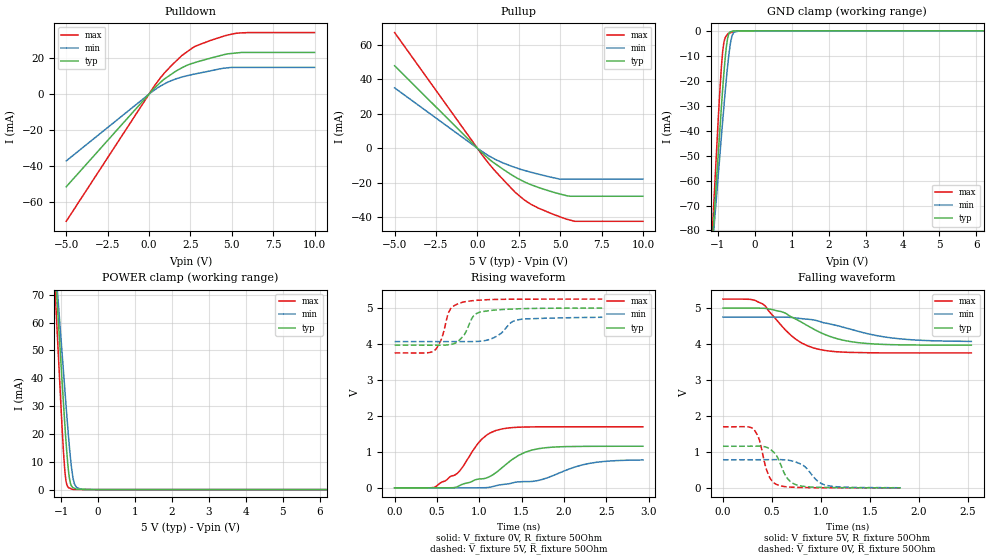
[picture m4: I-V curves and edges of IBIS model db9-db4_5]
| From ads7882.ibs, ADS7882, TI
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|   db9-db4_5 Model
[Model]   db9-db4_5
Model_type   3-state
Polarity   Non-Inverting
Enable   Active-Low
Vmeas = 2.5
Vref = 2.5
Cref = 20pF
Rref = 50
|   typ   min   max
|   (nom PVT)   (Fast PVT)   (slow PVT)
|C_comp from frequency sweep method (F=1.5MHz)
|Average
C_comp   1.143e-12   1.055e-12   1.239e-12
|ON state : BUFFER OUTPUT TURNED HIGH
|C_comp   1.109e-12   1.030e-12   1.196e-12
|OFF state: BUFFER IN HIGH IMPEDANCE
|C_comp   1.177e-12   1.080e-12   1.282e-12
|C_comp from LC tank measurement(L=1nH)
|Resonant Frequency(Hz)   6.030e+09   6.100e+09   5.860e+09
|C_comp   6.973e-13   6.814e-13   7.384e-13
|ON state : BUFFER OUTPUT TURNED HIGH
|Resonant Frequency(Hz)   6.030e+09   6.100e+09   5.860e+09
|C_comp   6.973e-13   6.814e-13   7.384e-13
|OFF state: BUFFER IN HIGH IMPEDANCE
|Resonant Frequency   6.000e+09   6.060e+09   5.330e+09
|C_comp   7.043e-13   6.905e-13   8.925e-13
| Where nom  PVT is Nominal Process,  5V,  25C
|   Fast PVT is Strong Process,   5.25V,  -40C
|   Slow PVT is Weak Process,   4.75V,  85C
[Voltage Range]   5   4.75   5.25
|Ambient Temperature   25   85   -40
|Junction Temperature
[Temperature Range]   25   85   -40
[Pullup Reference]   5   4.75   5.25
[Pulldown Reference]   0   0   0
[Power Clamp Reference]   5   4.75   5.25
[GND Clamp Reference]   0   0   0
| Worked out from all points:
|   slope of the pulldown table from 0 to 0.75 V, typ, clamps not added: 106 ohm
|   slope of the pullup table from 0 to 0.75 V, typ, clamps not added: 113 ohm
|   GND clamp passes 1 mA (typ) near -0.69 V on its own axis
|   POWER clamp passes 1 mA (typ) near -0.70 V on its own axis
|   falling waveform, V_fixture 5V, R_fixture 50Ohm: 20-80 % time 459ps typ, 622ps min, 331ps max; typ from 5 V to 3.97 V
|   rising waveform, V_fixture 0V, R_fixture 50Ohm: 20-80 % time 520ps typ, 769ps min, 344ps max; typ from 0 V to 1.16 V
|   rising waveform, V_fixture 5V, R_fixture 50Ohm: 20-80 % time 145ps typ, 189ps min, 117ps max; typ from 3.97 V to 5 V
|   falling waveform, V_fixture 0V, R_fixture 50Ohm: 20-80 % time 127ps typ, 163ps min, 98.5ps max; typ from 1.16 V to 0.001 V
[Pulldown]
|   Voltage   I(typ)   I(min)   I(max)
-5V       -51.38mA   -37.04mA   -70.55mA
307.8mV   3.159mA    2.15mA     4.364mA
927.3mV   8.407mA    5.669mA    11.73mA
1.982V    14.63mA    9.532mA    21.44mA
2.849V    17.78mA    11.34mA    26.81mA
4.505V    21.88mA    14.41mA    32.18mA
5.175V    22.77mA    14.84mA    33.67mA
6.004V    23.16mA    14.84mA    34.19mA
10V       23.16mA    14.84mA    34.19mA
[GND Clamp]
|   Voltage   I(typ)   I(min)   I(max)
-5V       -967.7mA   -803mA     -1.193A
-1.246V   -106.5mA   -104.5mA   -106.9mA
-1.029V   -57.47mA   -64.61mA   -45.63mA
-947mV    -39.41mA   -49.7mA    -23.63mA
-905mV    -30.17mA   -42.06mA   -14.11mA
-868.2mV  -22.67mA   -35.58mA   -7.769mA
-800mV    -10.28mA   -23.83mA   -2.63mA
-740mV    -3.15mA    -14.44mA   -1.388mA
-658.5mV  -390.9uA   -4.672mA   -764.2uA
-595mV    -43.54uA   -1.278mA   -477.3uA
-387.7mV  -28.37uA   -230.6nA   -2.849uA
10V       0A         0A         0A
[Pullup]
|   Voltage   I(typ)   I(min)   I(max)
-5V       47.7mA     34.91mA    66.9mA
370.8mV   -3.429mA   -2.455mA   -4.991mA
920mV     -7.931mA   -5.613mA   -11.48mA
1.353V    -10.83mA   -7.652mA   -16.11mA
2.276V    -16.6mA    -11.13mA   -25.44mA
2.849V    -19.51mA   -12.86mA   -30.04mA
3.694V    -22.7mA    -15.02mA   -34.67mA
4.961V    -26.4mA    -17.84mA   -39.56mA
5.595V    -27.78mA   -17.9mA    -41.55mA
5.878V    -27.78mA   -17.9mA    -42.27mA
10V       -27.78mA   -17.9mA    -42.27mA
[POWER Clamp]
|   Voltage   I(typ)   I(min)   I(max)
-5V       900mA      760.6mA    1.084A
-1.246V   96.38mA    96.53mA    92.6mA
-1.029V   50.17mA    58.28mA    35.81mA
-968mV    37.25mA    47.59mA    20.29mA
-899.8mV  23.1mA     35.62mA    6.524mA
-847.2mV  13.23mA    26.54mA    1.708mA
-795mV    5.774mA    17.98mA    656.1uA
-750mV    2.256mA    11.49mA    402.4uA
-695mV    815.8uA    5.464mA    92.38uA
-592mV    182.3uA    908.7uA    1.803uA
-373.5mV  115uA      14.55uA    892.3nA
10V       0A         0A         0A
[Ramp]
R_load = 50
|   typ   min   max
dV/dt_r   0.694817/5.19693e-10   0.469505/7.72354e-10   1.01975/3.43451e-10
dV/dt_f   0.618254/4.58969e-10   0.408899/6.31151e-10   0.897993/3.30611e-10
[Falling Waveform]
V_fixture = 5V
V_fixture_min = 4.75V
V_fixture_max = 5.25V
R_fixture = 50Ohm
|   Time   V(typ)   V(min)   V(max)
0s        5V         4.75V      5.25V
279.2ps   5V         4.75V      5.244V
392.5ps   4.997V     4.75V      5.132V
607.3ps   4.892V     4.748V     4.481V
716.8ps   4.731V     4.735V     4.192V
984.2ps   4.334V     4.631V     3.85V
1.222ns   4.11V      4.472V     3.777V
1.462ns   4.017V     4.297V     3.76V
1.894ns   3.976V     4.125V     3.754V
2.534ns   3.97V      4.074V     3.754V
[Rising Waveform]
V_fixture = 0V
V_fixture_min = 0V
V_fixture_max = 0V
R_fixture = 50Ohm
|   Time   V(typ)   V(min)   V(max)
0s        2.197nV    6.551nV    2.052nV
485ps     647.4uV    259uV      30.38mV
769.4ps   64.78mV    410.8uV    474.2mV
1.034ns   252.7mV    3.084mV    1.364V
1.16ns    361.9mV    37.19mV    1.56V
1.278ns   578.5mV    93.22mV    1.644V
1.462ns   901.1mV    166.1mV    1.686V
1.702ns   1.091V     210.3mV    1.697V
2.294ns   1.155V     677.5mV    1.698V
2.934ns   1.158V     776.1mV    1.699V
[Rising Waveform]
V_fixture = 5V
V_fixture_min = 4.75V
V_fixture_max = 5.25V
R_fixture = 50Ohm
|   Time   V(typ)   V(min)   V(max)
0s        3.969V     4.068V     3.753V
467.6ps   3.968V     4.068V     3.814V
553.7ps   3.969V     4.068V     4.14V
659.9ps   3.986V     4.068V     4.977V
806.6ps   4.212V     4.068V     5.166V
925.8ps   4.763V     4.069V     5.208V
1.024ns   4.9V       4.082V     5.225V
1.203ns   4.949V     4.215V     5.242V
1.459ns   4.981V     4.675V     5.248V
2.454ns   5V         4.745V     5.25V
[Falling Waveform]
V_fixture = 0V
V_fixture_min = 0V
V_fixture_max = 0V
R_fixture = 50Ohm
|   Time   V(typ)   V(min)   V(max)
0s        1.158V     782.7mV    1.7V
317.7ps   1.161V     783mV      1.615V
368ps     1.162V     783.6mV    1.361V
467.6ps   1.1V       784.8mV    333.9mV
565.1ps   799.8mV    786mV      74.64mV
666.7ps   232.8mV    771.2mV    26.55mV
765.9ps   69.68mV    694.7mV    12.89mV
967.4ps   16.9mV     184.4mV    3.943mV
1.073ns   10.62mV    61.29mV    1.939mV
1.814ns   929.8uV    3.688mV    1.177mV
